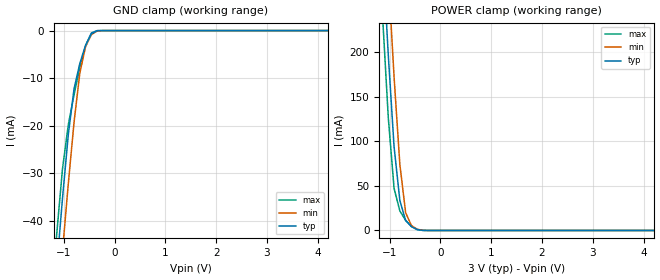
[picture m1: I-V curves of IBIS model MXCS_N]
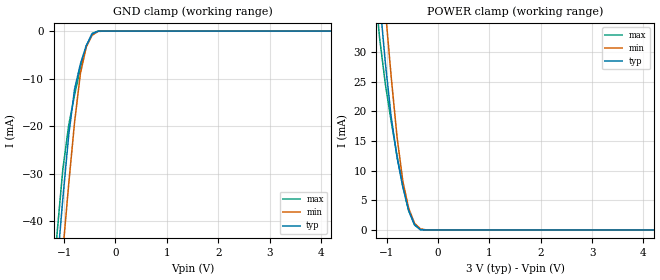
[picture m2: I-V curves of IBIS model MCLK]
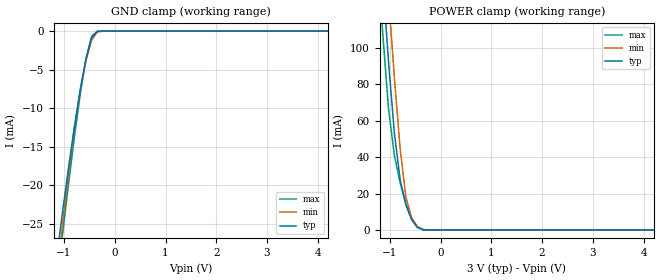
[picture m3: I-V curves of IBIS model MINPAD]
| Created by SiliconSmart  O-2018.09-SP2-3
[IBIS Ver]   4.0
[File Name]   as3101wa_rev1p4.ibs
[File Rev]   1.4
[Date]   Thursday Mar 21 2024
|[Source]   Avalanche Team
|[Notes]   Generated IBIS models from Silicon Smart
|[Rev 1.0]  Initial Release based on extracted netlist
|   Characterization
|[Rev 1.1]  Update the drive strength table for 3V
|[Rev 1.2]  Recharacterization of MIOPAD with Hspice run in high accuracy mode
|[Rev 1.3]  Recharacterization with Hspice to align with datasheet parameters
|[Rev 1.4]  Update the pin to the package pinout assignment
|[Disclaimer]   THE MODEL LIBRARIES ARE PROVIDED AS IS.
|[Copyright]   Copyright 2019, Avalanche Technology., All Rights Reserved
[Component]   AS30xx101_WSON
[Manufacturer] Avalanche Technology
| CONTENT :
| This file contains IBIS MODEL for PSRAM device
| AS3001101 AS3004101 AS3008101 AS3016101
| USAGE :
| The models are derived for the 2.7V to 3.6V I/O Operation.
| Temperatures for model generation: typ: 25, max: -40, min: 105
| Voltages : typ: 3.0V, min: 2.7V, max: 3.6V
| PACKAGES SUPPORTED :
| 8-pad WSON (5.0mm x 6.0mm)
| VERIFICATION
| Errors  : 0
| Warnings: 10
| All warnings due to non-monotonic data:
[Package]
|variable   typ   min   max
R_pkg   8.90E-04   8.89E-04  8.91E-04
L_pkg   1.185E-09  1.18E-09  1.19E-09
C_pkg   2.30E-13   2.21E-13  2.39E-13
[Pin]   signal_name   model_name   R_pin   L_pin   C_pin
1   CS#   MXCS_N   1.05E-01  1.35E-09  9.16E-14
2   SO   MIOPAD   1.05E-01  1.35E-09  9.16E-14
3   WP#   MINPAD   1.05E-01  1.35E-09  9.16E-14
5   SI   MINPAD   3.75E-02  3.89E-10  4.24E-14
6   CLK   MCLK   3.75E-02  3.89E-10  4.24E-14
7   HOLD#   MINPAD   3.75E-02  3.89E-10  4.24E-14
4   VSS   GND   NA   NA   NA
8   VCC   POWER   NA   NA   NA
[Model Selector] MIOPAD
| Model Description
M4_IOPAD_NVCR_OB03   45 Ohms drv strength
| Models and submodels in the file (4): MXCS_N (Input), MCLK (Input), MINPAD (Input), M4_IOPAD_NVCR_OB03 (Output)
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| XCS_N
[Model] MXCS_N
Model_type Input
Enable   Active-High
Vinl  =  0.9
Vinh  =  2.1
| Capacitance  typ   min   max
C_comp   3.070316e-12   2.808436e-12   3.350457e-12
| Variables   typ   min   max
[GND Clamp Reference]   0   0   0
[POWER Clamp Reference]   3   2.7   3.6
[Pulldown Reference]   0   0   0
[Pullup Reference]   3   2.7   3.6
[Temperature Range]   25   105   -40
[Voltage Range]   3   2.7   3.6
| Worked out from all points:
|   GND clamp passes 1 mA (typ) near -0.47 V on its own axis
|   POWER clamp passes 1 mA (typ) near -0.45 V on its own axis
[GND Clamp]
| Voltage   I(typ)   I(min)   I(max)
-3V       -315.1mA   -321.8mA   -312.6mA
-1.138V   -50.1mA    -61.4mA    -42.93mA
-1.024V   -35.38mA   -46.59mA   -29.17mA
-910.3mV  -22.01mA   -32.38mA   -19.91mA
-796.6mV  -12.29mA   -19.34mA   -13.52mA
-682.8mV  -6.93mA    -8.967mA   -7.783mA
-569mV    -3.073mA   -3.363mA   -3.169mA
-455.2mV  -632.4uA   -876.6uA   -499.8uA
-341.4mV  -24.5uA    -77.16uA   -7.616uA
-227.6mV  -421.5nA   -3.518uA   -35.99nA
6V        0A         0A         0A
[POWER Clamp]
| Voltage   I(typ)   I(min)   I(max)
-3V       2.46A      2.545A     2.395A
-1.138V   315.5mA    408mA      242.2mA
-1.024V   197.2mA    287.4mA    127mA
-910.3mV  94.22mA    172.8mA    47.4mA
-796.6mV  33.73mA    74.33mA    21.95mA
-682.8mV  11.27mA    20.05mA    11.43mA
-569mV    4.378mA    5.6mA      4.484mA
-455.2mV  1.088mA    1.361mA    987.1uA
-227.6mV  835.3nA    9.424uA    241.1nA
6V        0A         0A         0A
| CLK
[Model] MCLK
Model_type Input
Enable   Active-High
Vinl  =  0.9
Vinh  =  2.1
| Capacitance  typ   min   max
C_comp   2.706389e-12   2.515315e-12   2.914212e-12
| Variables   typ   min   max
[GND Clamp Reference]   0   0   0
[POWER Clamp Reference]   3   2.7   3.6
[Pulldown Reference]   0   0   0
[Pullup Reference]   3   2.7   3.6
[Temperature Range]   25   105   -40
[Voltage Range]   3   2.7   3.6
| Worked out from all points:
|   GND clamp passes 1 mA (typ) near -0.47 V on its own axis
|   POWER clamp passes 1 mA (typ) near -0.46 V on its own axis
[GND Clamp]
| Voltage   I(typ)   I(min)   I(max)
-3V       -312.9mA   -319.5mA   -311mA
-1.138V   -49.77mA   -60.97mA   -42.7mA
-1.024V   -35.15mA   -46.28mA   -29.02mA
-910.3mV  -21.89mA   -32.17mA   -19.81mA
-796.6mV  -12.24mA   -19.23mA   -13.45mA
-682.8mV  -6.904mA   -8.93mA    -7.747mA
-569mV    -3.064mA   -3.355mA   -3.158mA
-455.2mV  -631.5uA   -875.4uA   -499.1uA
-341.4mV  -24.5uA    -77.14uA   -7.616uA
-227.6mV  -421.5nA   -3.518uA   -35.99nA
6V        0A         0A         0A
[POWER Clamp]
| Voltage   I(typ)   I(min)   I(max)
-3V       249.7mA    259.7mA    242mA
-1.252V   50.97mA    61.19mA    43.36mA
-1.138V   39.14mA    48.99mA    32.5mA
-1.024V   28.15mA    37.13mA    24.58mA
-910.3mV  19.01mA    25.79mA    18.3mA
-796.6mV  12.24mA    15.66mA    12.48mA
-682.8mV  7.193mA    8.146mA    7.285mA
-569mV    3.26mA     3.629mA    3.179mA
-455.2mV  915uA      1.117mA    809.1uA
-341.4mV  55.3uA     196.8uA    44.86uA
-113.8mV  7.997nA    354.9nA    881.5pA
6V        0A         0A         0A
| INPAD
[Model] MINPAD
Model_type Input
Enable   Active-High
Vinl  =  0.9
Vinh  =  2.1
| Capacitance  typ   min   max
C_comp   3.872164e-12   3.590471e-12   4.177341e-12
| Variables   typ   min   max
[GND Clamp Reference]   0   0   0
[POWER Clamp Reference]   3   2.7   3.6
[Pulldown Reference]   0   0   0
[Pullup Reference]   3   2.7   3.6
[Temperature Range]   25   105   -40
[Voltage Range]   3   2.7   3.6
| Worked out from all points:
|   GND clamp passes 1 mA (typ) near -0.46 V on its own axis
|   POWER clamp passes 1 mA (typ) near -0.42 V on its own axis
[GND Clamp]
| Voltage   I(typ)   I(min)   I(max)
-3V       -145.8mA   -151.7mA   -144mA
-1.138V   -29.07mA   -31.55mA   -32.68mA
-1.024V   -23.24mA   -24.83mA   -26.15mA
-910.3mV  -17.69mA   -18.46mA   -19.83mA
-796.6mV  -12.47mA   -12.67mA   -13.82mA
-682.8mV  -7.718mA   -7.754mA   -8.316mA
-569mV    -3.663mA   -3.867mA   -3.675mA
-455.2mV  -839.2uA   -1.152mA   -666.1uA
-341.4mV  -35.63uA   -111.1uA   -11.17uA
-113.8mV  -8.642nA   -188.3nA   -1.888nA
6V        0A         0A         0A
[POWER Clamp]
| Voltage   I(typ)   I(min)   I(max)
-3V       949.8mA    984.2mA    923.5mA
-1.252V   183.6mA    221.4mA    154mA
-1.138V   136.7mA    174.2mA    107.6mA
-1.024V   92.09mA    128.1mA    66.35mA
-910.3mV  53.33mA    83.97mA    41.06mA
-796.6mV  27.72mA    44.75mA    25.94mA
-682.8mV  13.75mA    18.06mA    14.29mA
-569mV    5.664mA    6.605mA    5.738mA
-455.2mV  1.446mA    1.789mA    1.305mA
-341.4mV  77.09uA    287.6uA    62.73uA
-227.6mV  1.148uA    12.92uA    332nA
6V        0A         0A         0A
